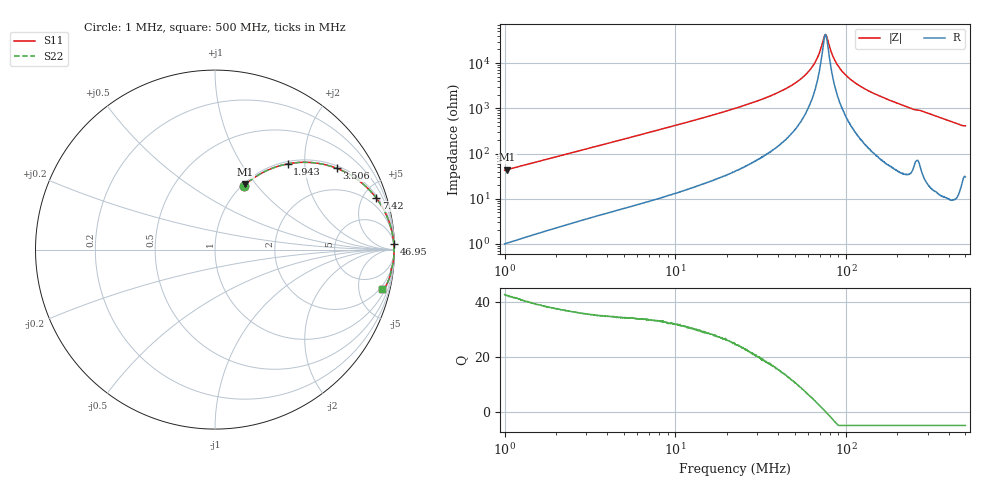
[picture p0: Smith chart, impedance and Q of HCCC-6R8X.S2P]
!s-Parameter Generated by FASTRON Sdn. Bhd.
!FASTRON P/N : HCCC-6R8X
!Keysight Technologies,E4991B,MY54100416,A.01.15
!Date: Thu Apr 02 15:51:25 2026
!Version  : Rev00 Thu Apr 02 15:51:25 2026
!Data & Calibration Information:
!PortZ  Port1:50+j0  Port2:50+j0
!When reading, reference impedance value at option line is always used.
!Remarks : This data is being provided solely for informational purposes.
!Freq	S11	S21	S12	S22
# Hz S dB R 50
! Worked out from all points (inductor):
!   1601 points, 1 MHz to 500 MHz, reference 50 ohm
!   read as one part in series: L = 6.76 uH near 1.032 MHz
!   highest Q = 42.2 at 1.036 MHz (marker M1), where L = 6.78 uH
!   self-resonance near 75.71 MHz
!   S11 on the Smith chart (normalised r, x): 1 MHz: 1.02, +0.85; 1.943 MHz: 1.04, +1.64; 3.506 MHz: 1.08, +2.94; 7.42 MHz: 1.19, +6.18; 46.95 MHz: 6, +61; 500 MHz: 1.61, -8.17
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1000000  -8.20 65.8  -0.80 -22.9  -0.80 -22.9  -8.20 65.8
1035575  -7.95 65.0  -0.85 -23.6  -0.85 -23.6  -7.95 65.0
1942909  -4.06 49.7  -2.35 -38.8  -2.35 -38.8  -4.06 49.7
2820919  -2.45 39.5  -3.93 -48.9  -3.93 -48.9  -2.45 39.5
3506344  -1.77 33.7  -5.11 -54.6  -5.11 -54.6  -1.77 33.7
7420238  -0.51 17.8  -10.31 -70.5  -10.31 -70.5  -0.51 17.8
7957584  -0.45 16.6  -10.86 -71.6  -10.86 -71.6  -0.45 16.6
2.236068e7  -0.08 5.7  -20.03 -82.0  -20.03 -82.0  -0.08 5.7
3.45472e7  -0.04 3.2  -24.95 -83.5  -24.95 -83.5  -0.04 3.2
4.695421e7  -0.03 1.9  -29.75 -83.4  -29.75 -83.4  -0.03 1.9
5.548932e7  -0.02 1.2  -33.60 -81.8  -33.60 -81.8  -0.02 1.2
6.307767e7  -0.02 0.7  -38.18 -78.2  -38.18 -78.2  -0.02 0.7
6.790877e7  -0.02 0.4  -42.34 -71.4  -42.34 -71.4  -0.02 0.4
7.396678e7  -0.02 0.1  -50.83 -35.0  -50.83 -35.0  -0.02 0.1
7.600545e7  -0.02 -0.0  -52.55 5.1  -52.55 5.1  -0.02 -0.0
7.779754e7  -0.02 -0.1  -50.76 35.9  -50.76 35.9  -0.02 -0.1
8.246482e7  -0.02 -0.3  -44.35 67.1  -44.35 67.1  -0.02 -0.3
8.639945e7  -0.02 -0.5  -40.92 74.9  -40.92 74.9  -0.02 -0.5
9.9366e7  -0.02 -1.0  -34.77 81.8  -34.77 81.8  -0.02 -1.0
1.254438e8  -0.02 -2.0  -29.13 84.3  -29.13 84.3  -0.02 -2.0
1.77937e8  -0.04 -3.7  -23.76 84.2  -23.76 84.2  -0.04 -3.7
5e8  -0.40 -13.4  -12.65 72.3  -12.65 72.3  -0.40 -13.4
